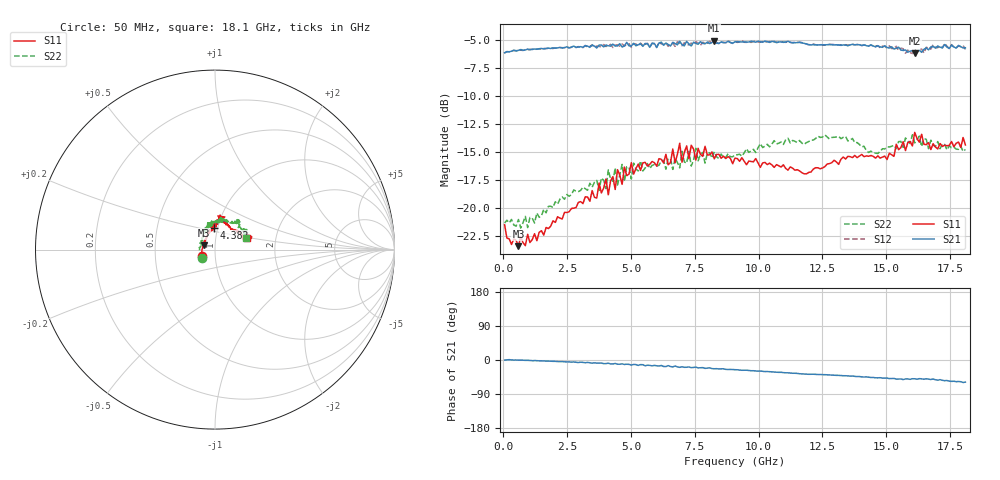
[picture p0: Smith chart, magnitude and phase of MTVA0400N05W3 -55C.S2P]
! Network Analyzer HP8720D.06.14 Serial No. US36140669
!  8 Jul 2005  06:27:29
! Frequency  S11  S21  S12  S22
# HZ  S  DB R 50
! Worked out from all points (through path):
!   201 points, 50 MHz to 18.1 GHz, reference 50 ohm
!   highest |S21| = -5.04 dB at 8.263 GHz (marker M1); lowest = -6.2 dB at 16.11 GHz (marker M2)
!   group delay of S21, straight-line fit = 9.36 ps
!   lowest |S11| = -23.4 dB at 591.5 MHz (marker M3), VSWR 1.14, Z = 44 + j2.1 ohm
!   |S11| at or under -10 dB: start of sweep to end of sweep
!   |S22| runs from -21.8 to -13.5 dB; largest |S21 - S12| = 0.025
!   S11 on the Smith chart (normalised r, x): 50 MHz: 0.86, -0.07; 4.382 GHz: 0.96, +0.24; 18.1 GHz: 1.42, +0.20
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5e7  -21.53 -153.0  -6.13 -0.2  -6.15 -0.0  -21.38 -147.2
5.915e8  -23.44 159.3  -5.92 -0.4  -5.90 -0.4  -21.05 164.2
3.1185e9  -19.63 105.7  -5.64 -6.3  -5.67 -6.7  -18.16 116.8
4.021e9  -17.43 97.0  -5.44 -9.5  -5.57 -8.3  -18.29 107.1
4.11125e9  -18.84 95.6  -5.50 -8.4  -5.50 -10.0  -16.61 105.6
4.382e9  -18.36 92.2  -5.53 -9.2  -5.45 -10.8  -16.44 105.5
4.47225e9  -16.59 87.2  -5.51 -11.1  -5.42 -9.4  -17.96 108.6
4.65275e9  -17.91 86.6  -5.61 -10.3  -5.35 -11.2  -16.12 106.5
4.743e9  -16.36 89.2  -5.52 -11.7  -5.53 -10.5  -17.66 102.3
5.104e9  -16.99 90.4  -5.28 -11.7  -5.33 -12.9  -16.01 96.8
6.09675e9  -15.61 82.7  -5.26 -15.9  -5.19 -15.6  -16.19 90.4
6.7285e9  -15.97 84.9  -5.31 -15.9  -5.56 -16.9  -15.55 81.7
6.909e9  -14.23 81.6  -5.10 -19.4  -5.26 -17.7  -16.43 79.8
6.99925e9  -15.92 81.0  -5.41 -17.8  -5.50 -19.7  -14.95 80.2
7.36025e9  -14.41 73.4  -5.52 -20.2  -5.27 -18.9  -16.27 83.0
7.54075e9  -15.73 74.6  -5.29 -18.7  -5.14 -21.1  -14.68 80.7
8.26275e9  -15.62 77.9  -5.04 -23.1  -5.22 -23.8  -15.00 67.8
9.075e9  -15.55 73.7  -5.16 -25.6  -5.13 -25.5  -15.27 63.0
1.21435e10  -16.54 50.3  -5.40 -37.5  -5.35 -37.6  -13.95 53.6
1.512175e10  -15.12 20.4  -5.71 -49.0  -5.52 -48.9  -14.56 39.4
1.61145e10  -13.26 19.1  -6.17 -49.5  -5.80 -49.9  -14.20 33.7
1.81e10  -14.38 20.3  -5.68 -58.4  -5.84 -58.3  -14.79 20.5
